FUNCTION "FC-callsLoader" : VOID
TITLE =Chiamata FC ABB
VERSION : 0.1

BEGIN
NETWORK
TITLE =Chiamata FC19 funzioni di allarme

      CALL "AlarmsLoader" ;
      NOP   0;
NETWORK
TITLE =Chiamata FC11 funzioni in manuale

      CALL "ManualLoader" ;
      NOP   0;
NETWORK
TITLE =Chiamata FC13 controllo elemento

      CALL "PartContr.Loader" ;
      NOP   0;
NETWORK
TITLE =Chiamata FC15 funzioni auto

      CALL "Auto/Cycle Loader" ;
      NOP   0;
NETWORK
TITLE =Chiamata FC16 funzioni valvole

      CALL "ValvesLoader" ;
      NOP   0;
NETWORK
TITLE =Chiamata FC17 funzioni segnali di uscita

      CALL "OutputsLoader" ;
      NOP   0;
NETWORK
TITLE =Chiamata FC20 funzioni di indicazione

      CALL "IndicationLoader" ;
      NOP   0;
END_FUNCTION

